| Texas Instruments Incorporated
| OCTAL BUFFER/DRIVER WITH 3-STATE OUTPUTS
| Marketing part#   Voltage Range   Package-type   #pins/pkg drawing
| SN74ALVC244DGV   1.65V - 3.6V   TVSOP   20-pin DGV
| SN74ALVC244DW   1.65V - 3.6V   SOIC   20-pin DW
| SN74ALVC244NS   1.65V - 3.6V   SOP   20-pin NS
| SN74ALVC244PW   1.65V - 3.6V   TSSOP   20-pin PW
| SN74ALVC244RGY   1.65V - 3.6V   VQFN   20-pin RGY
[IBIS Ver]   4.1
[File Name]   sn74alvc244.ibs
[File Rev]   1.2 | a_die
[Date]   January 20, 2016
[Source]   Data created from TI-SPICE simulations at TI-SLL.
   Texas Instruments Incorporated.
   Webench Design Center
   12500 TI Blvd
   Dallas, TX -75243
   For Support e-mail: elab_ibis@list.ti.com
[Notes]   Revision History
   Rev 1.2: 01/20/2016
   Rev 1.1: 05/03/2002
   -As there is no power clamp diode in the Input Models,
   we removed the Pwr Clamp table data from those Models.
   -The pulldown curves are affected by output feedback
   circuitrty.
[Disclaimer]  This model is designed as an aid for customers of Texas Instruments
 TI and its licensors and suppliers make no warranties, either expressed
 or implied, with respect to this  model, including the warranties of
 merchantability or fitness for a particular purpose.
 The model is provided solely on an "as is" basis. The entire risk as to
 its quality and performance is with the customer.
[Copyright] (C)Copyright 2016 Texas Instruments Incorporated.
   All rights reserved.
| Component ALVC244_DGV 20-pin TVSOP
[Component]   ALVC244_DGV
[Manufacturer]  Texas Instruments, Inc.
[Package]
|   typ   min   max
R_pkg   4.400e-02   3.800e-02   4.800e-02
L_pkg   2.561e-09   2.236e-09   2.961e-09
C_pkg   3.420e-13   2.640e-13   4.460e-13
[Pin]   signal_name   model_name   R_pin   L_pin   C_pin
1   1NOE   ALVC244_IN   4.400e-02   2.935e-09   4.170e-13
2   1A1   ALVC244_IN   4.200e-02   2.869e-09   4.460e-13
3   2Y4   ALVC244_OUT   4.300e-02   2.399e-09   3.160e-13
4   1A2   ALVC244_IN   4.400e-02   2.236e-09   2.650e-13
5   2Y3   ALVC244_OUT   4.600e-02   2.278e-09   2.640e-13
6   1A3   ALVC244_IN   4.500e-02   2.274e-09   2.640e-13
7   2Y2   ALVC244_OUT   4.400e-02   2.285e-09   2.690e-13
8   1A4   ALVC244_IN   4.300e-02   2.452e-09   3.200e-13
9   2Y1   ALVC244_OUT   4.400e-02   2.900e-09   4.460e-13
10   GND   GND   4.400e-02   2.961e-09   4.180e-13
11   2A1   ALVC244_IN   4.500e-02   2.954e-09   4.180e-13
12   1Y4   ALVC244_OUT   4.200e-02   2.847e-09   4.430e-13
13   2A2   ALVC244_IN   4.500e-02   2.453e-09   3.190e-13
14   1Y3   ALVC244_OUT   4.500e-02   2.297e-09   2.690e-13
15   2A3   ALVC244_IN   4.800e-02   2.334e-09   2.680e-13
16   1Y2   ALVC244_OUT   4.800e-02   2.335e-09   2.670e-13
17   2A4   ALVC244_IN   4.600e-02   2.299e-09   2.680e-13
18   1Y1   ALVC244_OUT   4.600e-02   2.457e-09   3.200e-13
19   2NOE   ALVC244_IN   4.300e-02   2.848e-09   4.410e-13
20   VCC   POWER   3.800e-02   2.812e-09   4.080e-13
| Component ALVC244_DW 20-pin SOIC
[Component]   ALVC244_DW
[Manufacturer]  Texas Instruments, Inc.
[Package]
|   typ   min   max
R_pkg   3.800e-02   3.300e-02   4.500e-02
L_pkg   5.012e-09   4.110e-09   6.349e-09
C_pkg   7.170e-13   5.300e-13   8.680e-13
[Pin]   signal_name   model_name   R_pin   L_pin   C_pin
1   1NOE   ALVC244_IN   4.200e-02   6.336e-09   8.650e-13
2   1A1   ALVC244_IN   4.300e-02   5.542e-09   8.670e-13
3   2Y4   ALVC244_OUT   3.400e-02   4.714e-09   7.320e-13
4   1A2   ALVC244_IN   3.400e-02   4.377e-09   5.910e-13
5   2Y3   ALVC244_OUT   3.600e-02   4.130e-09   5.330e-13
6   1A3   ALVC244_IN   3.500e-02   4.111e-09   5.300e-13
7   2Y2   ALVC244_OUT   3.400e-02   4.284e-09   5.830e-13
8   1A4   ALVC244_IN   3.400e-02   4.634e-09   7.260e-13
9   2Y1   ALVC244_OUT   4.000e-02   5.518e-09   8.650e-13
10   GND   GND   4.300e-02   6.349e-09   8.660e-13
11   2A1   ALVC244_IN   4.100e-02   6.281e-09   8.610e-13
12   1Y4   ALVC244_OUT   4.500e-02   5.561e-09   8.680e-13
13   2A2   ALVC244_IN   3.300e-02   4.778e-09   7.420e-13
14   1Y3   ALVC244_OUT   3.500e-02   4.414e-09   5.960e-13
15   2A3   ALVC244_IN   3.500e-02   4.110e-09   5.330e-13
16   1Y2   ALVC244_OUT   3.600e-02   4.130e-09   5.330e-13
17   2A4   ALVC244_IN   3.400e-02   4.377e-09   5.910e-13
18   1Y1   ALVC244_OUT   3.400e-02   4.714e-09   7.310e-13
19   2NOE   ALVC244_IN   4.300e-02   5.569e-09   8.680e-13
20   VCC   POWER   4.200e-02   6.308e-09   8.640e-13
| Component ALVC244_NS 20-pin SOP
[Component]   ALVC244_NS
[Manufacturer]  Texas Instruments, Inc.
[Package]
|   typ   min   max
R_pkg   4.400e-02   2.900e-02   5.800e-02
L_pkg   3.666e-09   2.317e-09   5.115e-09
C_pkg   5.480e-13   3.160e-13   7.250e-13
[Pin]   signal_name   model_name   R_pin   L_pin   C_pin
1   1NOE   ALVC244_IN   5.800e-02   5.115e-09   7.250e-13
2   1A1   ALVC244_IN   5.300e-02   4.591e-09   7.240e-13
3   2Y4   ALVC244_OUT   4.900e-02   3.754e-09   5.720e-13
4   1A2   ALVC244_IN   2.900e-02   2.549e-09   3.880e-13
5   2Y3   ALVC244_OUT   3.100e-02   2.317e-09   3.160e-13
6   1A3   ALVC244_IN   3.100e-02   2.317e-09   3.160e-13
7   2Y2   ALVC244_OUT   2.900e-02   2.556e-09   3.990e-13
8   1A4   ALVC244_IN   4.900e-02   3.754e-09   5.790e-13
9   2Y1   ALVC244_OUT   5.300e-02   4.591e-09   7.240e-13
10   GND   GND   5.800e-02   5.115e-09   7.250e-13
11   2A1   ALVC244_IN   5.800e-02   5.115e-09   7.250e-13
12   1Y4   ALVC244_OUT   5.300e-02   4.591e-09   7.240e-13
13   2A2   ALVC244_IN   4.900e-02   3.754e-09   5.790e-13
14   1Y3   ALVC244_OUT   2.900e-02   2.557e-09   3.990e-13
15   2A3   ALVC244_IN   3.100e-02   2.317e-09   3.160e-13
16   1Y2   ALVC244_OUT   3.100e-02   2.317e-09   3.160e-13
17   2A4   ALVC244_IN   2.900e-02   2.557e-09   3.990e-13
18   1Y1   ALVC244_OUT   4.900e-02   3.754e-09   5.790e-13
19   2NOE   ALVC244_IN   5.300e-02   4.591e-09   7.240e-13
20   VCC   POWER   5.800e-02   5.115e-09   7.250e-13
| Component ALVC244_PW 20-pin TSSOP
[Component]   ALVC244_PW
[Manufacturer]  Texas Instruments, Inc.
[Package]
|   typ   min   max
R_pkg   5.000e-02   4.200e-02   6.000e-02
L_pkg   2.802e-09   2.248e-09   3.553e-09
C_pkg   3.170e-13   2.020e-13   4.430e-13
[Pin]   signal_name   model_name   R_pin   L_pin   C_pin
1   1NOE   ALVC244_IN   5.500e-02   3.461e-09   4.400e-13
2   1A1   ALVC244_IN   5.500e-02   3.150e-09   4.010e-13
3   2Y4   ALVC244_OUT   4.200e-02   2.619e-09   3.020e-13
4   1A2   ALVC244_IN   4.500e-02   2.273e-09   2.020e-13
5   2Y3   ALVC244_OUT   4.500e-02   2.248e-09   2.240e-13
6   1A3   ALVC244_IN   4.500e-02   2.273e-09   2.260e-13
7   2Y2   ALVC244_OUT   4.400e-02   2.323e-09   2.050e-13
8   1A4   ALVC244_IN   4.600e-02   2.704e-09   3.070e-13
9   2Y1   ALVC244_OUT   6.000e-02   3.265e-09   4.110e-13
10   GND   GND   5.700e-02   3.506e-09   4.360e-13
11   2A1   ALVC244_IN   5.800e-02   3.553e-09   4.370e-13
12   1Y4   ALVC244_OUT   5.800e-02   3.193e-09   4.050e-13
13   2A2   ALVC244_IN   4.200e-02   2.704e-09   3.110e-13
14   1Y3   ALVC244_OUT   4.600e-02   2.392e-09   2.100e-13
15   2A3   ALVC244_IN   4.700e-02   2.334e-09   2.290e-13
16   1Y2   ALVC244_OUT   4.700e-02   2.300e-09   2.270e-13
17   2A4   ALVC244_IN   4.700e-02   2.349e-09   2.070e-13
18   1Y1   ALVC244_OUT   4.500e-02   2.677e-09   3.060e-13
19   2NOE   ALVC244_IN   6.000e-02   3.235e-09   4.060e-13
20   VCC   POWER   5.600e-02   3.487e-09   4.430e-13
| Component ALVC244_RGY 20-pin VQFN
[Component]   ALVC244_RGY
[Manufacturer]  Texas Instruments, Inc.
[Package]   | 20 pin VQFN RGY
|   typ   min   max
R_pkg   0.0969   0.0458   0.1182
L_pkg   1.4154n   1.0027n   1.7315n
C_pkg   0.1386p   0.1196p   0.1592p
[Pin]   signal_name   model_name   R_pin   L_pin   C_pin
1   1NOE   ALVC244_IN   0.08734   1.24640n   0.11957p
2   1A1   ALVC244_IN   0.11055   1.61673n   0.15067p
3   2Y4   ALVC244_OUT   0.10196   1.47947n   0.14411p
4   1A2   ALVC244_IN   0.09598   1.38443n   0.13711p
5   2Y3   ALVC244_OUT   0.09315   1.34070n   0.12663p
6   1A3   ALVC244_IN   0.09315   1.34060n   0.12663p
7   2Y2   ALVC244_OUT   0.09598   1.38423n   0.13711p
8   1A4   ALVC244_IN   0.10195   1.47927n   0.14411p
9   2Y1   ALVC244_OUT   0.11053   1.61643n   0.15073p
10   GND   GND   0.04579   1.00272n   0.15399p
11   2A1   ALVC244_IN   0.09422   1.35070n   0.12629p
12   1Y4   ALVC244_OUT   0.11819   1.73153n   0.15918p
13   2A2   ALVC244_IN   0.10809   1.56887n   0.15102p
14   1Y3   ALVC244_OUT   0.10013   1.44133n   0.14031p
15   2A3   ALVC244_IN   0.09667   1.38720n   0.13009p
16   1Y2   ALVC244_OUT   0.09336   1.33430n   0.12780p
17   2A4   ALVC244_IN   0.09360   1.33692n   0.13418p
18   1Y1   ALVC244_OUT   0.09727   1.39536n   0.13843p
19   2NOE   ALVC244_IN   0.10794   1.56632n   0.14939p
20   VCC   POWER   0.09131   1.30370n   0.12549p
| Model ALVC244_IN
[Model Selector]   ALVC244_IN
ALVC244_IN_18   1.8 volt Vcc
ALVC244_IN_25   2.5 volt Vcc
ALVC244_IN_33   3.3 volt Vcc
| Model ALVC244_OUT
[Model Selector]   ALVC244_OUT
ALVC244_OUT_18   1.8 volt Vcc
ALVC244_OUT_25   2.5 volt Vcc
ALVC244_OUT_33   3.3 volt Vcc
| Models and submodels in the file (6): ALVC244_IN_18 (Input), ALVC244_IN_25 (Input), ALVC244_IN_33 (Input), ALVC244_OUT_18 (3-state), ALVC244_OUT_25 (3-state), ALVC244_OUT_33 (3-state)
